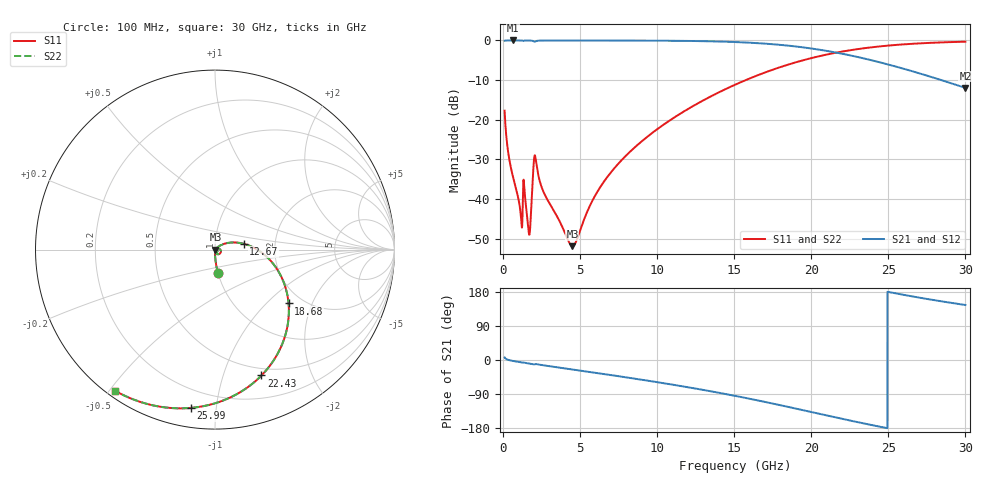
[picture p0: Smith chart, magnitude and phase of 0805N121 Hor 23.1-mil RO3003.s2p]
# GHz S MA R 50
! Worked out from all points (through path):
!   3201 points, 100 MHz to 30 GHz, reference 50 ohm
!   highest |S21| = -0.01 dB at 613.9 MHz (marker M1); lowest = -12.0 dB at 30 GHz (marker M2)
!   group delay of S21, straight-line fit = 20.9 ps
!   lowest |S11| = -51.8 dB at 4.501 GHz (marker M3), VSWR 1.01, Z = 50.2 - j0.117 ohm
!   |S11| at or under -10 dB: start of sweep to 15.74 GHz
!   |S22| runs from -51.8 to -0.3 dB; largest |S21 - S12| = 0
!   S11 on the Smith chart (normalised r, x): 100 MHz: 1.00, -0.26; 12.67 GHz: 1.37, +0.09; 18.68 GHz: 1.69, -1.37; 22.43 GHz: 0.42, -1.35; 25.99 GHz: 0.10, -0.85; 30 GHz: 0.02, -0.52
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0.1  0.1302 -82.9  0.9912 6.9  0.9912 6.9  0.1302 -82.9
0.361625  0.03569 -89.0  0.9987 0.0  0.9987 0.0  0.03569 -89.0
0.6139062  0.02016 -90.0  0.999 -2.3  0.999 -2.3  0.02016 -90.0
1.118469  0.00719 -83.5  0.9984 -5.9  0.9984 -5.9  0.00719 -83.5
1.426813  0.01062 -77.8  0.9963 -7.4  0.9963 -7.4  0.01062 -77.8
1.66975  0.00378 -46.2  0.9969 -9.2  0.9969 -9.2  0.00378 -46.2
1.781875  0.005198 11.7  0.9951 -10.1  0.9951 -10.1  0.005198 11.7
1.996781  0.0301 -1.2  0.9703 -11.5  0.9703 -11.5  0.0301 -1.2
2.11825  0.03188 -54.8  0.9768 -10.6  0.9768 -10.6  0.03188 -54.8
2.650844  0.01203 -87.9  0.9965 -14.2  0.9965 -14.2  0.01203 -87.9
4.500906  0.002559 -27.0  0.9973 -25.1  0.9973 -25.1  0.002559 -27.0
5.089563  0.004536 25.6  0.9971 -28.5  0.9971 -28.5  0.004536 25.6
6.90225  0.02063 42.2  0.9965 -39.2  0.9965 -39.2  0.02063 42.2
10.06978  0.07783 28.1  0.9926 -58.9  0.9926 -58.9  0.07783 28.1
12.66734  0.1623 11.6  0.9813 -76.6  0.9813 -76.6  0.1623 11.6
15.05  0.2764 -5.9  0.9544 -94.6  0.9544 -94.6  0.2764 -5.9
18.67537  0.508 -36.2  0.8527 -125.3  0.8527 -125.3  0.508 -36.2
20.03956  0.6011 -48.4  0.7898 -137.6  0.7898 -137.6  0.6011 -48.4
22.43156  0.7475 -69.7  0.6538 -159.0  0.6538 -159.0  0.7475 -69.7
25.01978  0.8619 -91.3  0.4957 179.4  0.4957 179.4  0.8619 -91.3
25.99153  0.8923 -98.7  0.4398 171.9  0.4398 171.9  0.8923 -98.7
30  0.964 -125.5  0.2522 145.1  0.2522 145.1  0.964 -125.5
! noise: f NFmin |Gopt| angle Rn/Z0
0.1  0.0004262  0.8589  0.6499  0.0006465
3.417  0.007029  0.7302  19.13  0.005049
6.743  0.0108  0.6723  37.1  0.005729
10.06  0.01504  0.6612  54.01  0.006811
13.39  0.01985  0.6684  69.79  0.007884
16.7  0.02568  0.6876  84.39  0.009014
20.03  0.03323  0.7162  98.09  0.0103
23.35  0.04356  0.7526  111.1  0.01185
26.67  0.05866  0.7955  123.8  0.01376
30  0.08235  0.8421  136.4  0.01596
